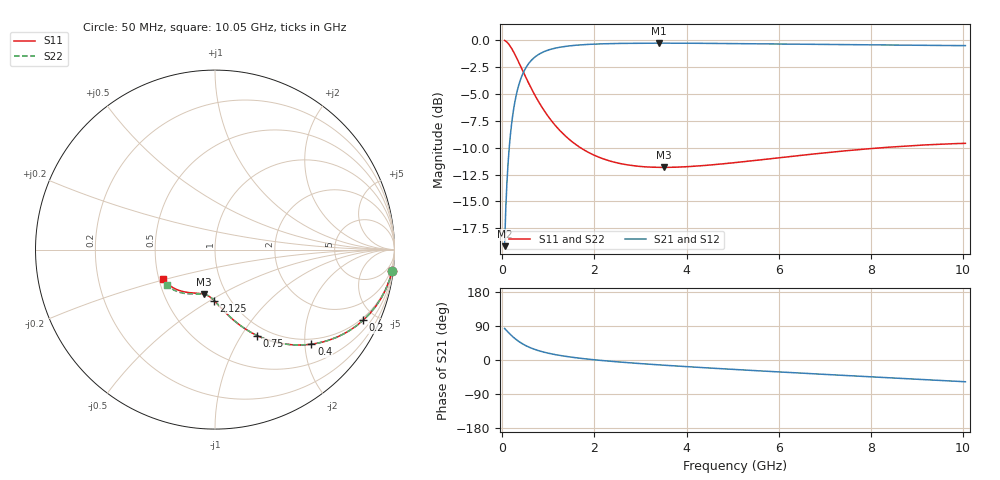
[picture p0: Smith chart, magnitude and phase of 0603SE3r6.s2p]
! AVX Thin Film Operation		Date: August 2001
! Description: Accu-P® Series, Thin Film, SMD, RF Capacitor
! Part Number: 06035J3R6ABT
! 50 MHz  -  10.05 GHz
! Serial Measurements
# mhz S db R 50
!	S11		S21		S12		S22
!	dB	Phase	dB	Phase	dB	Phase	dB	Phase
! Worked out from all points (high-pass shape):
!   401 points, 50 MHz to 10.05 GHz, reference 50 ohm
!   highest |S21| = -0.30 dB at 3.4 GHz (marker M1); lowest = -19.2 dB at 50 MHz (marker M2)
!   |S21| within 3 dB of the highest: 429.3 MHz to end of sweep
!   lowest |S11| = -11.8 dB at 3.5 GHz (marker M3), VSWR 1.69, Z = 39.3 - j20.9 ohm
!   |S11| at or under -10 dB: 1.692 GHz to 8.272 GHz (6.58 GHz wide, 132 % of centre)
!   |S22| runs from -11.8 to -0.1 dB; largest |S21 - S12| = 0
!   S11 on the Smith chart (normalised r, x): 50 MHz: 1, -17; 200 MHz: 0.88, -4.24; 400 MHz: 0.88, -2.14; 750 MHz: 0.88, -1.17; 2.125 GHz: 0.84, -0.52; 10.05 GHz: 0.53, -0.20
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50  -0.05 -6.7  -19.15 83.3  -19.15 83.3  -0.05 -6.7
100  -0.21 -13.3  -13.29 76.7  -13.29 76.7  -0.21 -13.3
125  -0.32 -16.5  -11.47 73.5  -11.47 73.5  -0.32 -16.5
150  -0.46 -19.6  -10.03 70.4  -10.03 70.4  -0.46 -19.6
200  -0.78 -25.5  -7.86 64.5  -7.86 64.5  -0.78 -25.5
250  -1.16 -30.9  -6.32 59.0  -6.32 59.0  -1.16 -30.9
300  -1.57 -35.9  -5.18 54.1  -5.18 54.1  -1.57 -35.9
400  -2.47 -44.5  -3.63 45.5  -3.63 45.5  -2.47 -44.5
575  -4.05 -55.8  -2.18 34.1  -2.18 34.1  -4.05 -55.8
750  -5.46 -63.9  -1.46 26.1  -1.46 26.1  -5.46 -63.9
925  -6.67 -69.9  -1.06 20.0  -1.06 20.0  -6.67 -69.9
1125  -7.82 -75.2  -0.79 14.7  -0.79 14.7  -7.82 -75.1
1375  -8.94 -80.3  -0.60 9.6  -0.60 9.6  -8.94 -80.2
1725  -10.09 -85.9  -0.45 4.1  -0.45 4.1  -10.09 -85.7
2125  -10.94 -91.0  -0.37 -0.9  -0.37 -0.9  -10.94 -90.6
2700  -11.59 -97.0  -0.32 -6.8  -0.32 -6.8  -11.59 -96.3
3400  -11.84 -103.2  -0.30 -12.9  -0.30 -12.9  -11.83 -102.1
3500  -11.84 -104.1  -0.30 -13.7  -0.30 -13.7  -11.83 -102.8
5050  -11.39 -116.0  -0.34 -25.1  -0.34 -25.1  -11.37 -113.6
6725  -10.61 -127.7  -0.41 -36.2  -0.41 -36.2  -10.58 -124.2
8400  -9.96 -139.0  -0.48 -46.9  -0.48 -46.9  -9.93 -134.2
10050  -9.60 -150.1  -0.53 -57.4  -0.53 -57.4  -9.56 -144.1
